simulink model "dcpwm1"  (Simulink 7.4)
settings: Solver=ode45  StartTime=0.0  StopTime=1.0  MaxStep=2e-4  RelTol=1e-4

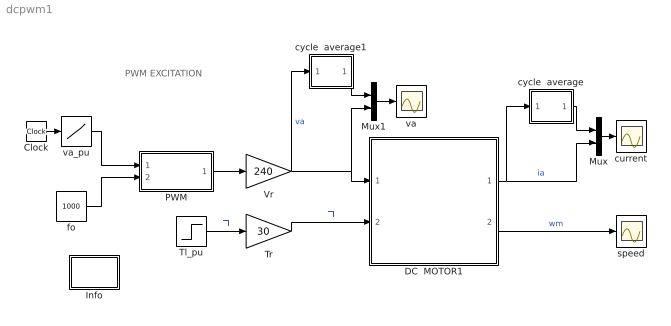
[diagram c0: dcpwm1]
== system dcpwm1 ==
  note: PWM EXCITATION
  Clock : Clock
  DC  MOTOR1 : Subsystem  mask{Ra=0.60, La=0.03, J=0.6, Bm=1e-5, K=1.85}
      mask prompts: Ra "Armature resistance [ohm]"; La "Armature inductance [H]"; J "Moment of inertia [Kg.m^2]"; Bm "Frictional torque cefficient"; K "Electromechanical coupling coefficient [N.m/A]"
      mask help: Block diagram of a dc motor. Inital conditions set for steady-state operation.
  Info : Subsystem
  Mux : Mux  Inputs=2
  Mux1 : Mux  Inputs=2
  PWM : Subsystem
  Tl_pu : Step  Time=0.1  Before=1  After=[.25 .50 .75 1.0]  SampleTime=0
  Tr : Gain  Gain=30  ParameterDataType=sfix(16)  ParameterScaling=2^0  OutDataType=sfix(16)  OutScaling=2^0
  Vr : Gain  Gain=240  ParameterDataType=sfix(16)  ParameterScaling=2^0  OutDataType=sfix(16)  OutScaling=2^0
  current : Scope
  cycle  average : Subsystem
  cycle  average1 : Subsystem
  fo : Constant  Value=1000  OutDataType=sfix(16)  OutScaling=2^0
  speed : Scope
  va : Scope
  va_pu : Lookup  InputValues=[0 0.5 0.5 2]  Table=[0.8 0.8 0.7 0.7]  OutDataType=sfix(16)  OutScaling=2^0
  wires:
  Vr/1 -> cycle  average1/1(sig), DC  MOTOR1/1(va), Mux1/2  "va"
  Tl_pu/1 -> Tr/1  "Tl"
  DC  MOTOR1/2(wm) -> speed/1  "wm"
  DC  MOTOR1/1(ia) -> cycle  average/1(sig), Mux/2  "ia"
  cycle  average/1(ave) -> Mux/1
  Mux/1 -> current/1
  Clock/1 -> va_pu/1
  PWM/1(Output) -> Vr/1
  fo/1 -> PWM/2(frequency)
  va_pu/1 -> PWM/1(control)
  Tr/1 -> DC  MOTOR1/2(Tl)  "Tl"
  cycle  average1/1(ave) -> Mux1/1
  Mux1/1 -> va/1

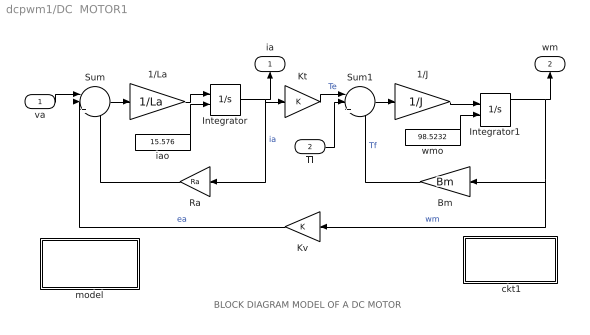
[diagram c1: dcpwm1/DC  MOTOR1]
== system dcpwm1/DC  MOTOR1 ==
  note: BLOCK DIAGRAM MODEL OF A DC MOTOR
  va : Inport  OutDataType=sfix(16)  OutScaling=2^0
  Tl : Inport  Port=2  OutDataType=sfix(16)  OutScaling=2^0
  " ckt1" : Subsystem
  1/J : Gain  Gain=1/J  ParameterDataType=sfix(16)  ParameterScaling=2^0  OutDataType=sfix(16)  OutScaling=2^0
  1/La : Gain  Gain=1/La  ParameterDataType=sfix(16)  ParameterScaling=2^0  OutDataType=sfix(16)  OutScaling=2^0
  Bm : Gain  Gain=Bm  ParameterDataType=sfix(16)  ParameterScaling=2^0  OutDataType=sfix(16)  OutScaling=2^0
  Integrator : Integrator  InitialConditionSource=external  InitialCondition=16.2162
  Integrator1 : Integrator  InitialConditionSource=external  InitialCondition=98.5245
  Kt : Gain  Gain=K  ParameterDataType=sfix(16)  ParameterScaling=2^0  OutDataType=sfix(16)  OutScaling=2^0
  Kv : Gain  Gain=K  ParameterDataType=sfix(16)  ParameterScaling=2^0  OutDataType=sfix(16)  OutScaling=2^0
  Ra : Gain  Gain=Ra  ParameterDataType=sfix(16)  ParameterScaling=2^0  OutDataType=sfix(16)  OutScaling=2^0
  Sum : Sum  Inputs=||+--  OutDataType=sfix(16)  OutScaling=2^0
  Sum1 : Sum  Inputs=||+--  OutDataType=sfix(16)  OutScaling=2^0
  iao : Constant  Value=15.576  OutDataType=sfix(16)  OutScaling=2^0
  model : Subsystem
  wmo : Constant  Value=98.5232  OutDataType=sfix(16)  OutScaling=2^0
  ia : Outport
  wm : Outport  Port=2
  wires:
  Kv/1 -> Sum/2  "ea"
  Ra/1 -> Sum/3
  Kt/1 -> Sum1/1  "Te"
  Bm/1 -> Sum1/3  "Tf"
  Sum/1 -> 1/La/1
  1/La/1 -> Integrator/1
  Integrator/1 -> Ra/1, Kt/1, ia/1  "ia"
  Sum1/1 -> 1/J/1
  1/J/1 -> Integrator1/1
  Integrator1/1 -> Bm/1, Kv/1, wm/1  "wm"
  va/1 -> Sum/1
  Tl/1 -> Sum1/2
  iao/1 -> Integrator/2
  wmo/1 -> Integrator1/2

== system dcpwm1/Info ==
  note: This demo simulates the running of a DC motor with PWM (unipolar) excitation (5 hp 240V 1200 rpm) rated torque Tr = 30 N.m

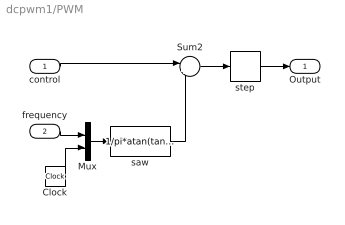
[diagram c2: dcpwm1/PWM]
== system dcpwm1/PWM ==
  control : Inport  OutDataType=sfix(16)  OutScaling=2^0
  frequency : Inport  Port=2  OutDataType=sfix(16)  OutScaling=2^0
  Clock : Clock
  Mux : Mux  Inputs=2
  Sum2 : Sum  Inputs=|+-  OutDataType=sfix(16)  OutScaling=2^0
  saw : Fcn  Expr=1/pi*atan(tan((2*pi*u(1)*u(2)-pi)/2))+0.5
  step : Relay  OutDataType=sfix(16)  OutScaling=2^0
  Output : Outport
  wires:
  Clock/1 -> Mux/2
  Mux/1 -> saw/1
  control/1 -> Sum2/1
  frequency/1 -> Mux/1
  saw/1 -> Sum2/2
  step/1 -> Output/1
  Sum2/1 -> step/1

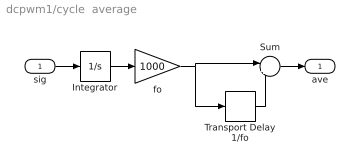
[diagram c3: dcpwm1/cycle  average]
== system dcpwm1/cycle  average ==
  sig : Inport  OutDataType=sfix(16)  OutScaling=2^0
  Integrator : Integrator
  Sum : Sum  Inputs=|+-  OutDataType=sfix(16)  OutScaling=2^0
  Transport Delay 1/fo : TransportDelay  DelayTime=1/1000
  fo : Gain  Gain=1000  ParameterDataType=sfix(16)  ParameterScaling=2^0  OutDataType=sfix(16)  OutScaling=2^0
  ave : Outport
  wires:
  Integrator/1 -> fo/1
  fo/1 -> Sum/1, Transport Delay 1/fo/1
  sig/1 -> Integrator/1
  Transport Delay 1/fo/1 -> Sum/2
  Sum/1 -> ave/1

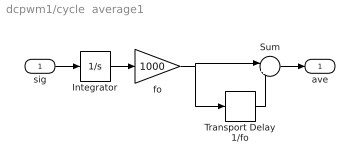
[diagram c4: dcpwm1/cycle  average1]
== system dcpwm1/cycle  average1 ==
  sig : Inport  OutDataType=sfix(16)  OutScaling=2^0
  Integrator : Integrator
  Sum : Sum  Inputs=|+-  OutDataType=sfix(16)  OutScaling=2^0
  Transport Delay 1/fo : TransportDelay  DelayTime=1/1000
  fo : Gain  Gain=1000  ParameterDataType=sfix(16)  ParameterScaling=2^0  OutDataType=sfix(16)  OutScaling=2^0
  ave : Outport
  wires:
  Integrator/1 -> fo/1
  fo/1 -> Sum/1, Transport Delay 1/fo/1
  sig/1 -> Integrator/1
  Transport Delay 1/fo/1 -> Sum/2
  Sum/1 -> ave/1

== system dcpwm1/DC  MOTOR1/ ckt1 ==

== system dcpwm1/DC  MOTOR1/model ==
  note: Electrical system equation: va = Ra.ia + La.dia/dt + ea where ea = K.wm Mechanical system equation: Te = J.dwm/dt + Tl.signum(wm) + f(wm) where Te = K.ia
  note: Mathematical model of the dc machine
